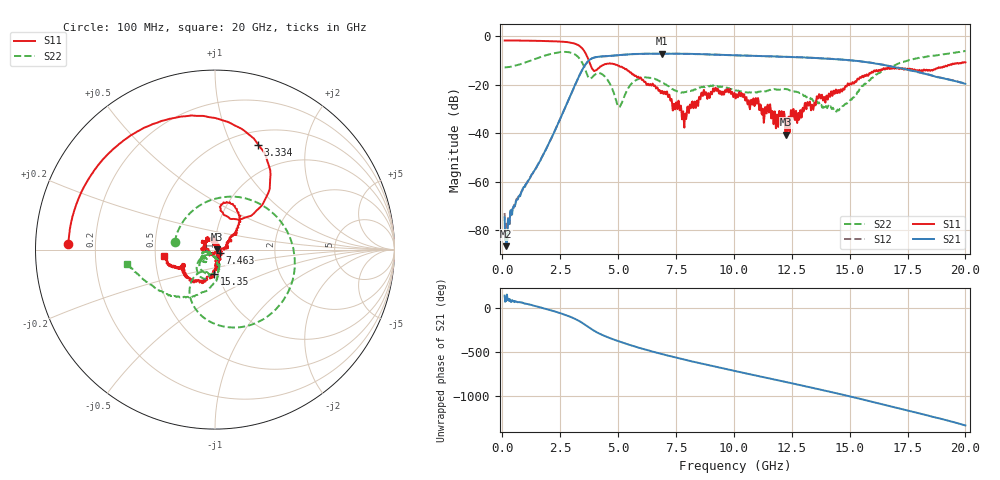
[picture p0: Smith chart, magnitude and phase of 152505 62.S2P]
!  2-Port S-parameters saved by WinCal
! VAR MeasName=S-Parameters (CALIBRATED_DATA) read from VNA (N5230C)
! VAR MeasDate=4/10/2015 9:35:06 AM
! VAR NAME=152505 62
! VAR FILENAME=152505 62.S2P
! VAR DATE=4/10/2015 9:35:06 AM
! VAR PHYS_PORTS=1,2
# Hz S DB R 50
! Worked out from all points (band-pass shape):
!   801 points, 100 MHz to 20 GHz, reference 50 ohm
!   highest |S21| = -7.17 dB at 6.891 GHz (marker M1); lowest = -86.6 dB at 174.6 MHz (marker M2)
!   |S21| within 3 dB of the highest: 3.721 GHz to 15.28 GHz (11.56 GHz wide, 122 % of centre)
!   lowest |S11| = -40.5 dB at 12.24 GHz (marker M3), VSWR 1.02, Z = 50.9 + j0.221 ohm
!   |S11| at or under -10 dB: 3.733 GHz to end of sweep
!   |S22| runs from -31.1 to -6.0 dB; largest |S21 - S12| = 0.005
!   S11 on the Smith chart (normalised r, x): 100 MHz: 0.10, +0.02; 3.334 GHz: 0.65, +1.27; 7.463 GHz: 1.05, -0.04; 15.35 GHz: 0.95, -0.26; 20 GHz: 0.55, -0.04
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1e8  -1.75 177.6  -74.68 145.1  -72.89 33.7  -12.88 169.8
1.74625e8  -1.75 175.9  -86.57 84.4  -79.40 28.6  -12.81 162.0
1.269125e9  -1.87 149.2  -56.99 37.4  -57.01 36.0  -9.85 65.4
2.23925e9  -2.09 121.3  -39.56 -33.9  -39.62 -34.3  -6.97 -7.5
3.33375e9  -3.99 67.6  -16.10 -147.7  -16.15 -147.4  -9.20 -108.4
3.43325e9  -4.82 59.5  -14.22 -163.6  -14.23 -163.3  -10.63 -118.3
4.104875e9  -13.60 77.8  -8.52 81.9  -8.52 82.1  -15.29 -109.2
5.050125e9  -12.22 57.6  -7.76 -20.1  -7.80 -20.2  -29.28 -109.6
5.72175e9  -16.40 38.8  -7.32 -77.8  -7.38 -77.8  -18.46 -85.8
6.741625e9  -22.42 30.9  -7.19 -153.5  -7.20 -153.7  -18.28 -135.8
6.890875e9  -22.57 15.0  -7.17 -163.9  -7.20 -163.8  -19.01 -138.3
7.463e9  -30.18 -32.7  -7.20 157.9  -7.20 157.8  -22.32 -140.0
7.861e9  -37.66 -89.6  -7.27 132.2  -7.24 132.5  -23.09 -129.8
8.632125e9  -24.13 -178.3  -7.41 84.7  -7.41 84.6  -20.96 -129.0
1.005e10  -24.21 121.4  -7.85 1.1  -7.88 1.0  -22.43 -151.2
1.2239e10  -40.54 13.3  -8.48 -123.6  -8.50 -124.2  -21.79 -159.8
1.338325e10  -28.24 -52.6  -8.93 169.5  -8.90 169.7  -25.91 -167.3
1.450262e10  -22.22 -80.8  -9.56 102.0  -9.52 102.0  -30.39 -122.8
1.534838e10  -17.47 -92.4  -10.22 49.2  -10.25 49.0  -22.86 -80.2
1.669162e10  -13.14 -128.1  -12.26 -37.7  -12.25 -38.4  -12.81 -99.8
1.838312e10  -14.22 -152.5  -15.76 -148.9  -15.75 -148.7  -8.30 -143.0
2e10  -10.80 -173.1  -19.62 97.6  -19.63 98.0  -6.04 -170.7
